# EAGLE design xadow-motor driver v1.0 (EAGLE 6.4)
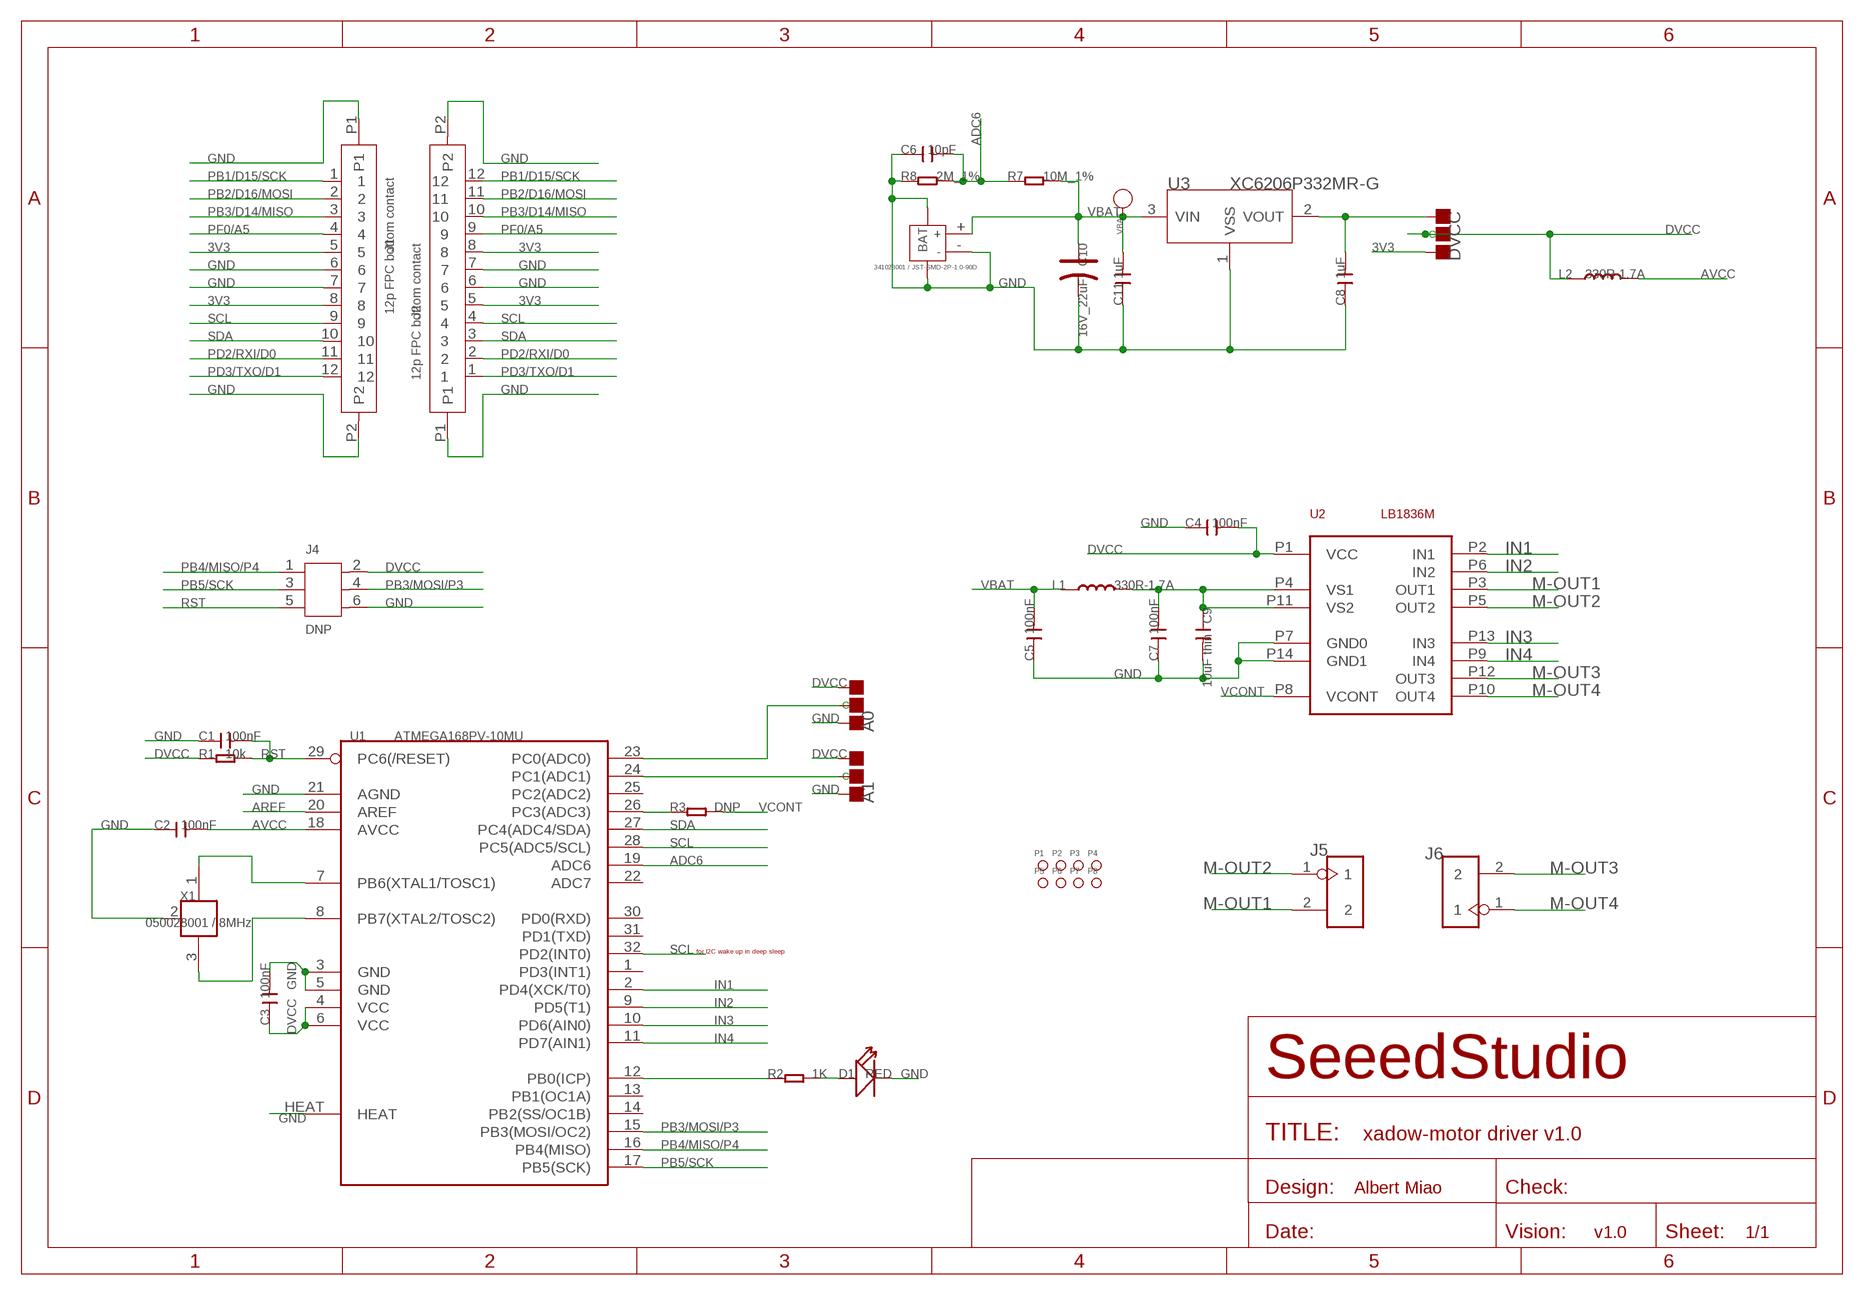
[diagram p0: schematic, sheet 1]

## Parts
A0  DNP  PAD-JUMPER-3P-40*40  [3P-SMD-4.1X1.5]
A1  DNP  PAD-JUMPER-3P-40*40  [3P-SMD-4.1X1.5]
BAT  341023001 / JST-SMD-2P-1.0-90D  JACK-JST-2P-SMD-PW'1.0'  [JST-SMD-2P-1.0-90D]
C1  100nF  C-0603  [C0603]
C2  100nF  C-0603  [C0603]
C3  100nF  C-0603  [C0603]
C4  100nF  C-0603  [C0603]
C5  100nF  C-0603  [C0603]
C6  10pF  C-0603  [C0603]
C7  100nF  C-0603  [C0603]
C8  1uF  C-0603  [C0603]
C9  10uF thin  C-0805  [C0805]
C10  16V_22uF  CAP-AVX-A  [AVX-A]
C11  1uF  C-0603  [C0603]
D1  RED  LED'0603'  [LED-0603]
DVCC  DNP  PAD-JUMPER-3P-40*40  [3P-SMD-4.1X1.5]
J1  12p FPC bottom contact  FPC052002-12LT  [12P-0.5]
J2  12p FPC bottom contact  FPC052002-12LT  [12P-0.5]
J4  DNP  HEADER-2X3P-1.27  [2X3P-1.27]
J5  HEADER-2P-2.0  [2P-2.0]
J6  HEADER-2P-2.0  [2P-2.0]
L1  330R-1.7A  L'0603'  [L0603]
L2  330R-1.7A  L'0603'  [L0603]
P1  PAD-MARK  [ROUND-MARK-1.0]
P2  PAD-MARK  [ROUND-MARK-1.0]
P3  PAD-MARK  [ROUND-MARK-1.0]
P4  PAD-MARK  [ROUND-MARK-1.0]
P5  PAD-MARK  [ROUND-MARK-1.0]
P6  PAD-MARK  [ROUND-MARK-1.0]
P7  PAD-MARK  [ROUND-MARK-1.0]
P8  PAD-MARK  [ROUND-MARK-1.0]
R1  10k  R-0603  [R0603]
R2  1K  R-0603  [R0603]
R3  DNP  R-0603  [R0603]
R7  10M_1%  R-0603  [R0603]
R8  2M_1%  R-0603  [R0603]
U1  ATMEGA168PV-10MU  MEGA8  [MLF32X]
U2  LB1836M  [MFP14S]
U3  XC6206P332MR-G  XC6206MR  [SOT23]
VBAT  PAD-TEST-POINT'4545'  [TP_4545]
X1  050028001 / 8MHz  XTAL_NCVER  [XTAL_3X2]

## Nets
3V3: DVCC.11(R) J1.5 J1.8 J2.5 J2.8
ADC6: C6.2 R7.1 R8.2 U1.19(ADC6)
AREF: U1.20(AREF)
AVCC: C2.2 L2.2 U1.18(AVCC)
DVCC [vcc]: A0.00(L) A1.00(L) C3.1 C4.2 DVCC.MM(C) J4.2 L2.1 R1.1 U1.4(VCC) U1.6(VCC) U2.P1(VCC)
GND: A0.11(R) A1.11(R) BAT.3 BAT.4 BAT.- C1.1 C2.1 C3.2 C4.1 C5.1 C6.1 C7.1 C8.1 C9.2 C10.- C11.1 D1.- J1.6 J1.7 J1.P1 J1.P2 J2.6 J2.7 J2.P1 J2.P2 J4.6 R8.1 U1.3(GND) U1.5(GND) U1.21(AGND) U1.HEAT U2.P7(GND0) U2.P14(GND1) U3.1(VSS) X1.2(GND)
IN1: U1.2(PD4(XCK/T0)) U2.P2(IN1)
IN2: U1.9(PD5(T1)) U2.P6(IN2)
IN3: U1.10(PD6(AIN0)) U2.P13(IN3)
IN4: U1.11(PD7(AIN1)) U2.P9(IN4)
M-OUT1 [HighCur]: J5.2 U2.P3(OUT1)
M-OUT2 [HighCur]: J5.1 U2.P5(OUT2)
M-OUT3 [HighCur]: J6.2 U2.P12(OUT3)
M-OUT4 [HighCur]: J6.1 U2.P10(OUT4)
N$2 [vcc]: C7.2 C9.1 L1.2 U2.P4(VS1) U2.P11(VS2)
N$3: R2.1 U1.12(PB0(ICP))
N$4: R3.1 U1.26(PC3(ADC3))
N$6: C8.2 DVCC.00(L) U3.2(VOUT)
N$7: A0.MM(C) U1.23(PC0(ADC0))
N$8: A1.MM(C) U1.24(PC1(ADC1))
N$9: D1.+ R2.2
N$22: U1.7(PB6(XTAL1/TOSC1)) X1.1
N$26: U1.8(PB7(XTAL2/TOSC2)) X1.3
PB1/D15/SCK: J1.1 J2.12
PB2/D16/MOSI: J1.2 J2.11
PB3/D14/MISO: J1.3 J2.10
PB3/MOSI/P3: J4.4 U1.15(PB3(MOSI/OC2))
PB4/MISO/P4: J4.1 U1.16(PB4(MISO))
PB5/SCK: J4.3 U1.17(PB5(SCK))
PD2/RXI/D0: J1.11 J2.2
PD3/TXO/D1: J1.12 J2.1
PF0/A5: J1.4 J2.9
RST: C1.2 J4.5 R1.2 U1.29(PC6(/RESET))
SCL: J1.9 J2.4 U1.28(PC5(ADC5/SCL)) U1.32(PD2(INT0))
SDA: J1.10 J2.3 U1.27(PC4(ADC4/SDA))
VBAT [vcc]: BAT.+ C5.2 C10.+ C11.2 L1.1 R7.2 U3.3(VIN) VBAT.T
VCONT: R3.2 U2.P8(VCONT)
Unconnected: U1.1(PD3(INT1)) U1.13(PB1(OC1A)) U1.14(PB2(SS/OC1B)) U1.22(ADC7) U1.25(PC2(ADC2)) U1.30(PD0(RXD)) U1.31(PD1(TXD))

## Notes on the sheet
- for I2C wake up in deep sleep
- Albert Miao
- v1.0

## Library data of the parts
A0 A1 DVCC = Discrete:PAD-JUMPER-3P; PARTNO: DNP
BAT = Connector :JACK-JST-2P-SMD-PW
C1-C9 C11 = Discrete:C*: Ceramic Capacitors
C10 = Discrete:CAP*: Electrolytic Capacitors,Tantalum Capacitors and Super Capacitors
D1 = Discrete:LED*
J1 J2 = template:FPC052002-12LT
J4 = template:HEADER-2X3P-1.27
J5 J6 = Connector:HEADER-2P
L1 L2 = Discrete:L*
P1-P8 = Discrete:PAD-MARK; PARTNO: DNP
R1-R3 R7 R8 = Discrete:R*
U1 = ICs_v54:MEGA8
U2 = LeoBuild:LB1836M
U3 = IC:XC6206: LOW ESR Cap.Compatible Positive Voltage Regulators
VBAT = Discrete:PAD-TEST-POINT; PARTNO: DNP
X1 = CPT_SMD:XTAL_NC

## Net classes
0 default: width 0.152 mm, drill 0.305 mm, clearance 0.152 mm
1 vcc: width 0.203 mm
2 HighCur: width 0.203 mm

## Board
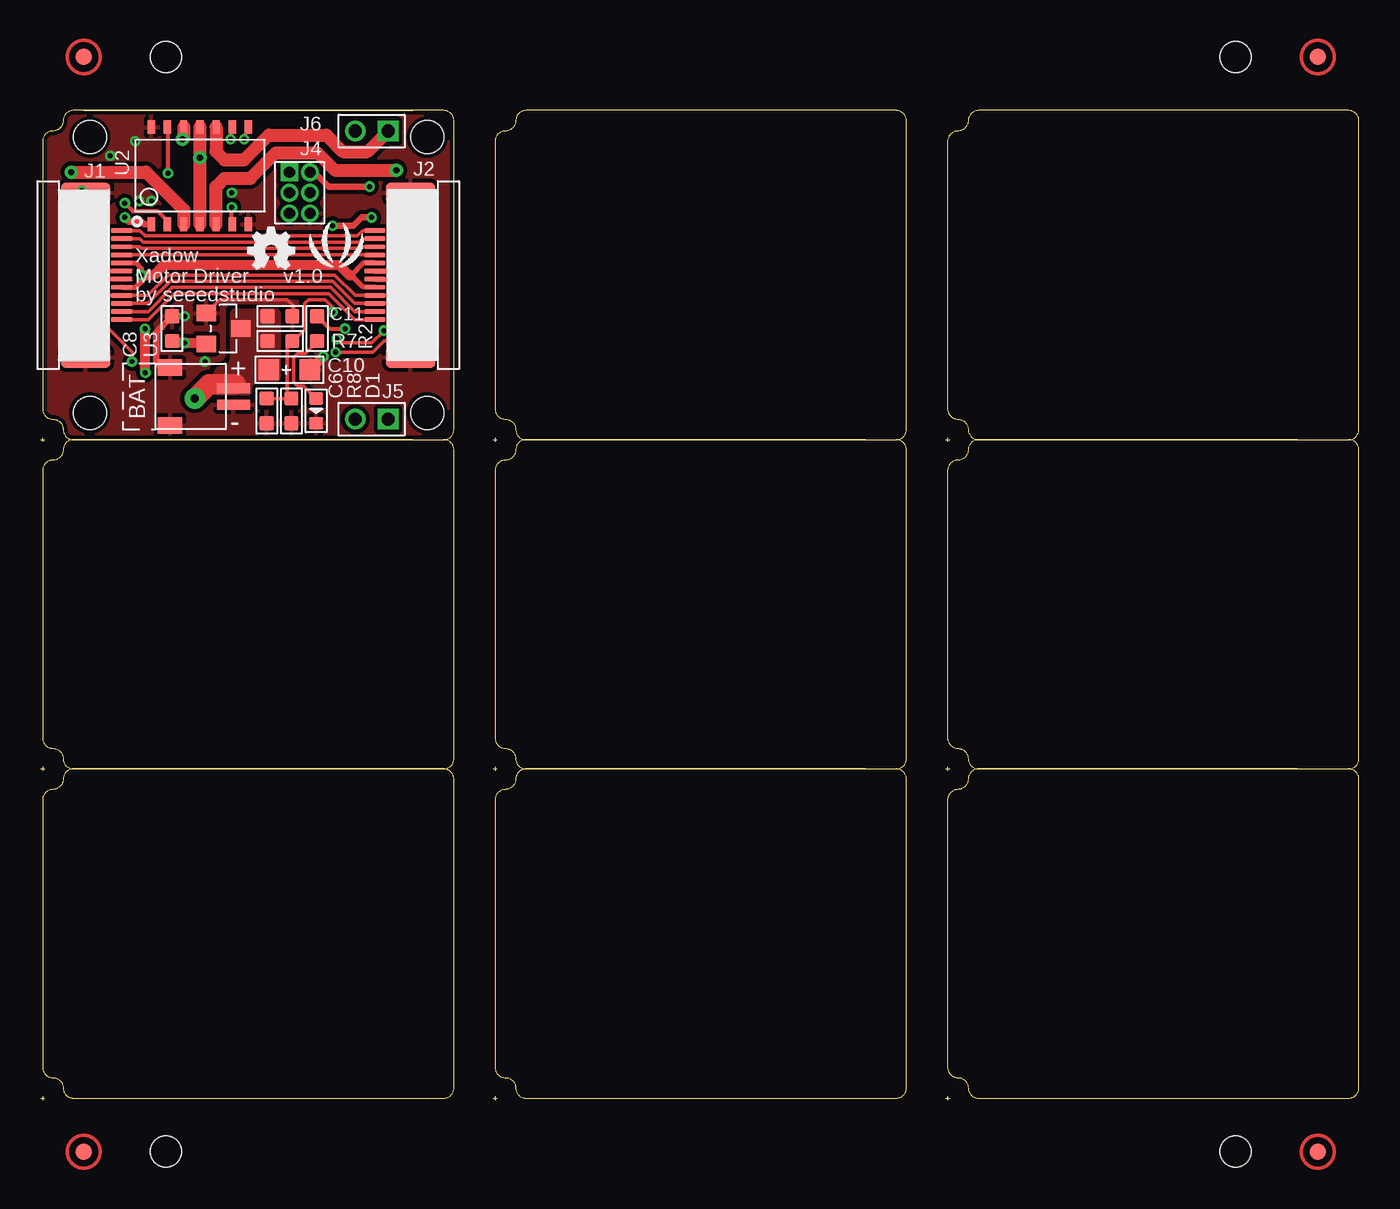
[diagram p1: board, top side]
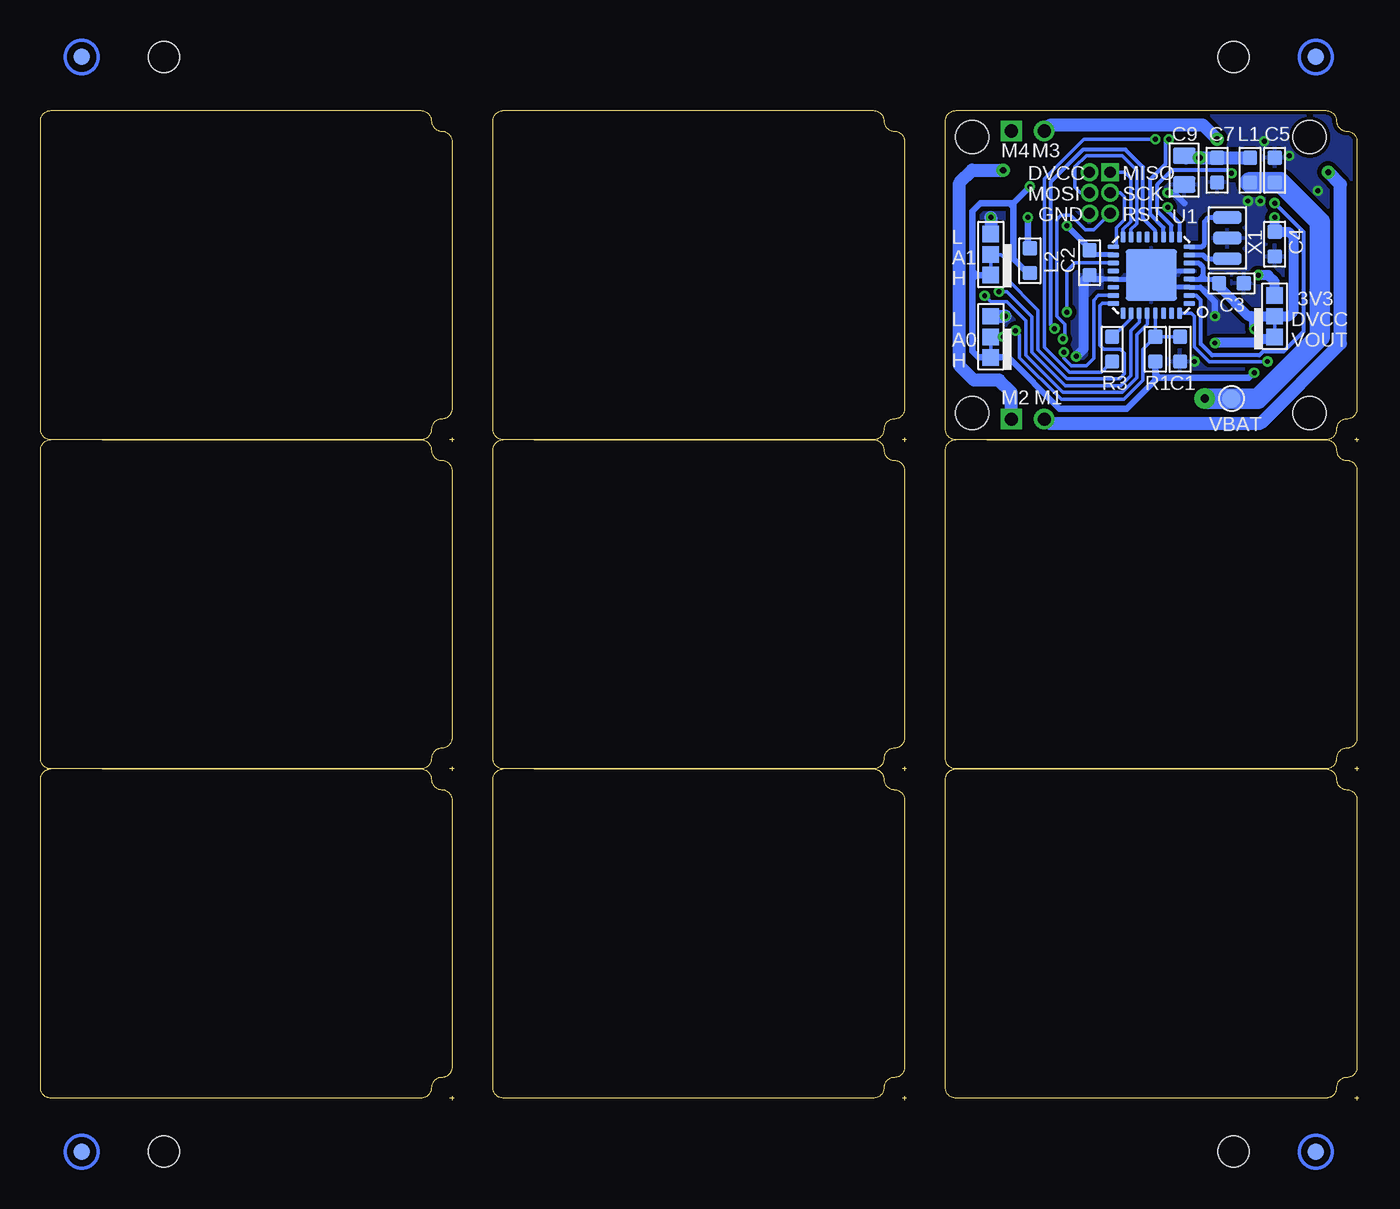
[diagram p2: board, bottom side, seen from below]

Size 81.41 x 61.09 mm. Coordinates in mm from the lower left corner, seen from the top.
Outline: 161 segments
Copper layers (1*16): Top 0.035mm / dielectric 1.5mm / Bottom 0.035mm
Design rules "SeeedStudio_rule_no_angle_090911 *": minimum track width 6mil, minimum drill 12mil, track to track 6mil, track to pad 6mil, pad to pad 6mil, via to via 6mil, smd to smd 0mil, copper to edge 10mil, drill to drill 10mil, minimum pad ring 6mil, minimum via ring 6mil, stop-mask expansion 2mil, vias tented up to drill 25mil, thermal gap 10mil
Holes 2.03 mm at 3.05,42.42 3.05,59.44 23.88,59.44 23.88,42.42
Holes 1.91 mm at 73.79,64.39 7.75,64.39 7.75,-3.17 73.79,-3.17
tRestrict: area 20,50.9 to 21.3,51; area 4.4,50.9 to 5.7,51; 12 lines
bRestrict: 12 lines

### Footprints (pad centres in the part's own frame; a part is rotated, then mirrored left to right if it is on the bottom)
3P-SMD-4.1X1.5 = smd 1.016 x 1.016: 00 -1.27,0; 11 1.27,0; MM 0,0
JST-SMD-2P-1.0-90D = smd 1.524 x 1.016: 3 -3.429,1.778; 4 -3.429,-1.778 | smd 2.032 x 0.635: + 0.508,0.508; - 0.508,-0.508
C0603 = smd 0.889 x 0.889: 1 -0.762,0; 2 0.762,0
C0805 = smd 1.016 x 1.397: 1 -0.889,0; 2 0.889,0
AVX-A = smd 1.27 x 1.27: + -1.27,0; - 1.27,0
LED-0603 = smd 0.762 x 0.889: + -0.762,0; - 0.762,0
12P-0.5 = smd 0.3 x 1.3: 1 -2.75,2.35; 2 -2.25,2.35; 3 -1.75,2.35; 4 -1.25,2.35; 5 -0.75,2.35; 6 -0.25,2.35; 7 0.25,2.35; 8 0.75,2.35; 9 1.25,2.35; 10 1.75,2.35; 11 2.25,2.35; 12 2.75,2.35 | smd 1.27 x 3.048: P1 -5.08,0.127; P2 5.08,0.127
2X3P-1.27 = drill 0.686 pad 1.092 square: 1 -0.635,1.27 | drill 0.686 pad 1.092: 2 0.635,1.27; 3 -0.635,0; 4 0.635,0; 5 -0.635,-1.27; 6 0.635,-1.27
2P-2.0 = drill 0.813 pad 1.27 square: 1 -1.016,0 | drill 0.813 pad 1.27: 2 1.016,0
L0603 = smd 0.889 x 0.889: 1 -0.762,0; 2 0.762,0
ROUND-MARK-1.0 = smd 1.016 x 1.016: P$1 0,0
R0603 = smd 0.889 x 0.889: 1 -0.762,0; 2 0.762,0
MLF32X = smd 0.7 x 0.3: 1 -2.35,1.75; 2 -2.35,1.25; 3 -2.35,0.75; 4 -2.35,0.25; 5 -2.35,-0.25; 6 -2.35,-0.75; 7 -2.35,-1.25; 8 -2.35,-1.75; 17 2.35,-1.75; 18 2.35,-1.25; 19 2.35,-0.75; 20 2.35,-0.25; 21 2.35,0.25; 22 2.35,0.75; 23 2.35,1.25; 24 2.35,1.75 | smd 0.3 x 0.7: 9 -1.75,-2.35; 10 -1.25,-2.35; 11 -0.75,-2.35; 12 -0.25,-2.35; 13 0.25,-2.35; 14 0.75,-2.35; 15 1.25,-2.35; 16 1.75,-2.35; 25 1.75,2.35; 26 1.25,2.35; 27 0.75,2.35; 28 0.25,2.35; 29 -0.25,2.35; 30 -0.75,2.35; 31 -1.25,2.35; 32 -1.75,2.35 | smd 3.175 x 3.175: HEAT 0,0
MFP14S = smd 0.45 x 0.85: P1 1,-0.8; P2 2,-0.8; P3 3,-0.8; P4 4,-0.8; P5 5,-0.8; P6 6,-0.8; P7 7,-0.8; P8 7,5.2; P9 6,5.2; P10 5,5.2; P11 4,5.2; P12 3,5.2; P13 2,5.2; P14 1,5.2
SOT23 = smd 1.016 x 1.2: 1 -0.95,-1.06; 2 0.95,-1.06; 3 0,1.06
TP_4545 = smd 1.143 x 1.143: T 0,0
XTAL_3X2 = smd 0.762 x 1.778: 1 -1.27,0; 2 0,0; 3 1.27,0

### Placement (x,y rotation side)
A0  22.73,47.12 90 bottom
A1  22.73,52.2 90 bottom
BAT  11.43,43.43 0 top
C1  11.05,46.35 90 bottom
C2  16.64,51.69 90 bottom
C3  7.87,50.42 0 bottom
C4  5.21,52.83 90 bottom
C5  5.21,57.4 270 bottom
C6  13.97,42.55 90 top
C7  8.76,57.4 90 bottom
C8  8.13,47.62 270 top
C9  10.79,57.4 270 bottom
C10  15.37,45.09 0 top
C11  14.8,48.39 180 top
D1  17.02,42.55 270 top
DVCC  5.21,48.39 90 bottom
J1  2.67,50.93 270 top
J2  22.99,50.93 90 top
J4  16,56.01 0 top
J5  20.45,42.04 180 top
J6  20.45,59.82 180 top
L1  6.73,57.4 90 bottom
L2  20.32,51.82 90 bottom
P1  not placed on the board
P2  not placed on the board
P3  not placed on the board
P4  not placed on the board
P5  not placed on the board
P6  not placed on the board
P7  not placed on the board
P8  not placed on the board
R1  12.57,46.35 90 bottom
R2  17.08,47.62 270 top
R3  15.24,46.35 270 bottom
R7  14.8,46.86 180 top
R8  15.49,42.55 90 top
U1  12.83,50.93 180 bottom
U2  5.84,54.86 0 top
U3  11.3,47.62 270 top
U$2  [SMALL_SEEED_LOGO]  18.29,52.96 0 top
U$3  [OSHW_FILLX100_NOTEXT]  12.83,51.31 0 top
VBAT  7.87,43.31 0 bottom
X1  8.13,53.21 90 bottom

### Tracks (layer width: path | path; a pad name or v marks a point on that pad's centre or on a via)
3V3  (via drill 0.3 pad 0.64)
  Top 0.305: J1.8 5.87,50.18 6.22,50.53 v6.22,50.93 6.22,51.33 5.87,51.68 J1.5 | J2.8 19.93,51.68 19.18,50.93 19.93,50.18 J2.5
  Top 0.61: v6.22,50.93 6.99,50.93 7.62,51.56 18.41,51.56 19.05,50.93 19.18,50.93
  Bottom 0.61: DVCC.11 5.21,50.55 5.59,50.93 v6.22,50.93
ADC6  (via drill 0.3 pad 0.64)
  Top 0.203: C6.2 R8.2 15.49,43.43 15.24,43.69 15.24,46.55 R7.1 15.62,46.86 16.32,47.56 16.32,49.17 16.55,49.4 17.58,49.4 18.03,48.95 v18.03,48.64
  Bottom 0.203: U1.19 17.54,51.68 18.03,51.18 v18.03,48.64
AVCC  (via drill 0.3 pad 0.64)
  Top 0.406: v18.03,53.98 19.3,53.98 19.81,54.48 v20.45,54.48
  Bottom 0.305: U1.18 16.36,52.18 C2.2
  Bottom 0.406: C2.2 16.64,52.58 v18.03,53.98 | v20.45,54.48 20.45,52.7 L2.2
DVCC  (via drill 0.3 pad 0.64)
  Top 0.406: J4.2 16.89,57.28 17.78,56.39 v20.32,56.39 | U2.P1 6.39,54.06 6.22,54.23 5.46,54.23 v5.21,54.48
  Top 0.61: v6.45,47.6 6.44,47.59 6.44,44.93 v6.48,44.89
  Bottom 0.203: A0.00 22.73,47.12 | A1.00 22.73,52.2 | DVCC.MM 5.21,47.12
  Bottom 0.254: 9.4,50.67 9.65,50.93 9.91,50.67
  Bottom 0.305: 10.02,51.68 U1.6 9.89,51.68 9.65,51.44 9.65,50.93 9.65,50.68 | U1.4 9.65,50.68 | 9.65,50.68 8.89,50.68 C3.1
  Bottom 0.406: R1.1 12.57,44.83 | 12.57,44.83 12.57,44.58 | 12.57,44.58 12.57,44.45 14.34,42.69 18.49,42.69 21.65,45.85 A0.00 23.49,45.85 23.88,46.23 23.88,50.67 | 12.57,44.58 12.32,44.58 | L2.1 20.45,51.05 21.34,51.94 21.34,55.12 | 23.88,50.67 23.88,50.93 | 23.88,50.93 23.88,51.18 | 23.88,51.18 23.88,54.86 23.37,55.37 21.59,55.37 | 21.34,55.12 21.34,55.37 | 21.34,55.37 v20.32,56.39 | 21.59,55.37 21.34,55.37 | 21.59,55.37 21.34,55.12 | A1.00 23.62,50.93 | 23.62,50.93 23.88,50.93 | 12.32,44.58 12.57,44.83 | 12.32,44.58 6.79,44.58 v6.48,44.89 | 23.62,50.93 23.88,51.18 | 23.62,50.93 23.88,50.67
  Bottom 0.61: DVCC.MM 5.32,48.39 5.33,48.39 | v5.21,54.48 C4.2 4.35,53.59 4.06,53.31 4.06,48.64 4.32,48.39 DVCC.MM | C3.1 8.64,50.19 6.83,48.39 6.67,48.39 | 6.67,48.39 6.35,48.39 | 6.35,48.39 6.22,48.39 | 6.22,48.39 5.33,48.39 DVCC.MM | v6.45,47.6 6.45,48.16 | 6.45,48.17 6.45,48.28 6.35,48.39 | 6.45,48.16 6.22,48.39 | 6.45,48.16 6.45,48.17 | 6.45,48.17 6.67,48.39
GND  (via drill 0.3 pad 0.64)
  Top 0.203: U3.1 11.07,49.4 15.24,49.4 15.62,49.02 15.62,48.45 C11.1
  Top 0.305: J1.6 3.18,51.18 | J1.7 3.18,50.68 3.18,50.67 | J2.6 21.47,50.68 21.84,51.05 22.73,51.05 | J2.7 21.33,51.18 21.72,51.56 22.61,51.56
  Top 0.406: 7.62,45.09 7.15,45.56 7.15,47.41 C8.1
  Top 0.61: C10.- 16.76,45.09 16.76,45.21 17.4,45.85
  Bottom 0.305: 15.87,50.68 U1.21 12.95,50.68 12.83,50.8 | 12.83,50.8 12.83,50.55 12.46,50.18 U1.3 9.79,50.18 9.53,49.91 | 12.83,50.8 U1.HEAT 12.83,51.18 12.82,51.18 U1.5
  Bottom 0.406: 15.87,50.68 16.39,50.68 C2.1 | 9.53,49.91 8.89,49.28 v8.89,48.39 | v11.81,56.01 11.43,56.01 10.79,55.37
  Bottom 0.61: C2.1 17.02,50.55 17.02,46.35 v17.46,45.91
  Bottom 0.813: A0.11 v21.84,48.39 | v22.73,54.48 A1.11
  other vias: 10.16,45.59 5.84,59.18 4.32,58.29 6.1,55.5 6.86,55.5 2.54,56.13
  pour Top (isolate 0.254, rank 2): 0.13,61.09 25.53,61.09 25.53,40.77 0.13,40.77
  pour Bottom (isolate 0.254, rank 2): 0.13,61.09 25.53,61.09 25.53,40.77 0.13,40.77
IN1  (via drill 0.3 pad 0.64)
  Top 0.254: U2.P2 7.84,54.26 7.24,54.86 5.71,54.86 v5.21,55.37
  Bottom 0.254: U1.2 10.07,49.68 9.78,49.38 9.78,46.69 9.07,45.97 6.16,45.97 5.93,46.21 4.66,46.21 3.43,47.44 3.43,53.59 v5.21,55.37
IN2  (via drill 0.3 pad 0.64)
  Top 0.203: 11.81,54.09 U2.P6
  Top 0.254: 11.81,54.09 v11.81,55.12
  Bottom 0.254: U1.9 11.08,54.13 11.81,54.86 v11.81,55.12
IN3  (via drill 0.3 pad 0.64)
  Top 0.254: U2.P13 7.84,57.25 v7.87,57.21
  Bottom 0.254: U1.10 11.58,53.99 12.44,54.85 12.44,56.52 11.56,57.4 8.06,57.4 v7.87,57.21
IN4  (via drill 0.3 pad 0.64)
  Top 0.203: v11.75,59.31 11.75,59.97 U2.P9
  Bottom 0.254: U1.11 12.08,53.86 12.89,54.67 12.89,56.83 11.94,57.78 11.94,59.12 v11.75,59.31
M-OUT1  (via drill 0.38 pad 0.81)
  Top 0.813: v1.9,57.28 6.52,57.28 8.84,54.95 U2.P3
  Bottom 0.813: J5.2 19.18,41.78 6.07,41.78 1.14,46.71 1.14,56.52 v1.9,57.28
M-OUT2  (via drill 0.38 pad 0.81)
  Top 0.813: U2.P5 10.84,56.39 11.35,56.9 12.95,56.9 14.53,58.48 17.09,58.48 18.16,57.4 v21.97,57.4
  Bottom 0.813: v21.97,57.4 23.88,57.4 24.67,56.61 24.67,45.35 23.77,44.45 22.23,44.45 21.46,43.69 J5.1
M-OUT3  (via drill 0.38 pad 0.81)
  Top 0.813: U2.P12 8.84,59.39 v8.76,59.31
  Bottom 0.813: v8.76,59.31 9.65,60.2 19.05,60.2 J6.2
M-OUT4
  Top 0.813: U2.P10 10.84,58.55 11.35,58.04 12.57,58.04 14.1,59.56 17.65,59.56 18.67,58.55 20.19,58.55 J6.1
N$2  (via drill 0.38 pad 0.81)
  Top 0.813: U2.P11 v9.84,58.17 U2.P4
  Bottom 0.813: L1.2 C7.2 v9.84,58.17 10.67,58.17 C9.1
N$3  (via drill 0.3 pad 0.64)
  Top 0.203: R2.1 17.27,48.39
  Top 0.254: R2.1 17.84,47.62 v18.8,47.62
  Bottom 0.254: U1.12 12.58,53.66 13.34,54.42 13.34,57.6 14.41,58.67 17.04,58.67 19.05,56.66 19.05,47.88 v18.8,47.62
N$4
  Bottom 0.203: R3.1 15.19,47.12 14.08,48.23 U1.26
N$6  (via drill 0.3 pad 0.64)
  Top 0.61: 10.24,46.53 U3.2 10.18,46.74 v8.89,46.74 8.25,46.74 C8.2
  Bottom 0.61: v8.89,46.74 6.22,46.74 5.97,46.99 5.33,46.99 DVCC.00
N$7  (via drill 0.3 pad 0.64)
  Top 0.203: v21.97,47.12 21.72,46.86 21.21,46.86 20.51,46.16 v18.22,46.16
  Bottom 0.203: v21.97,47.12 A0.MM | U1.23 16.09,49.68 16.38,49.38 16.38,45.79 16.85,45.33 17.77,45.33 18.22,45.78 v18.22,46.16
N$8
  Bottom 0.203: A1.MM 22.1,52.2 21.84,51.94 21.84,50.8 19.81,48.77 19.81,46.32 18.03,44.53 14.78,44.53 14.48,44.83 14.48,46.1 14.73,46.35 15.75,46.35 16,46.61 16,49.02 15.85,49.18 U1.24
N$9
  Top 0.203: D1.+ 16.26,44.07 15.88,44.07 15.62,44.32 15.62,45.85 15.88,46.1 16.38,46.1 17.02,46.74 17.02,46.8 R2.2
N$22
  Bottom 0.305: U1.7 9.63,52.18 9.4,51.94 X1.1
N$26
  Bottom 0.305: U1.8 9.68,52.68 9.53,52.83 9.53,54.23 9.27,54.48 X1.3
PB1/D15/SCK
  Top 0.203: J1.1 6.14,53.68 6.48,53.34 19.56,53.34 19.89,53.68 J2.12
PB2/D16/MOSI
  Top 0.203: J1.2 6.13,53.18 6.35,52.96 19.68,52.96 19.9,53.18 J2.11
PB3/D14/MISO
  Top 0.203: J1.3 6.12,52.68 6.22,52.58 19.81,52.58 19.91,52.68 J2.10
PB3/MOSI/P3
  Bottom 0.203: U1.15 14.08,53.74 13.72,54.1 13.72,57.4 14.61,58.29 16.84,58.29 17.53,57.6 17.53,56.34 17.2,56.01 J4.4
PB4/MISO/P4
  Bottom 0.203: U1.16 14.58,53.75 14.1,54.23 14.1,56.9 14.48,57.28 J4.1
PB5/SCK
  Bottom 0.203: J4.3 14.73,56.01 14.48,55.75 14.48,54.36 14.99,53.85 14.99,52.87 U1.17
PD2/RXI/D0
  Top 0.203: J1.11 6.64,48.68 8.13,50.16 17.91,50.16 19.39,48.68 J2.2
PD3/TXO/D1
  Top 0.203: J1.12 6.65,48.18 8.25,49.78 17.78,49.78 19.39,48.18 J2.1
PF0/A5
  Top 0.203: J1.4 J2.9
RST  (via drill 0.3 pad 0.64)
  Top 0.203: v18.29,46.99 18.54,46.74 20.45,46.74 v21.21,47.5
  Bottom 0.203: C1.2 R1.2 | R1.2 13.34,46.35 13.34,44.45 14.53,43.26 18.38,43.26 20.95,45.83 20.95,47.24 v21.21,47.5 | U1.29 R1.2 | J4.5 16.38,53.72 16.89,53.72 17.78,54.61 18.41,54.61 18.67,54.36 18.67,48.39 18.16,47.88 18.16,47.12 v18.29,46.99
SCL  (via drill 0.3 pad 0.64)
  Top 0.203: v23.11,49.66 23.11,50.19 22.76,50.55 21.95,50.55 21.59,50.19 21.59,49.84 21.42,49.68 J2.4 19.41,49.68 18.16,50.93 7.87,50.93 6.62,49.68 J1.9 4.21,49.68 3.99,49.45 3.99,47.83 5.65,46.16 v5.65,45.59
  Bottom 0.203: U1.32 10.35,48.58 10.16,48.39 10.16,46.51 9.24,45.59 v5.65,45.59 | U1.28 13.08,47.88 13.72,47.24 13.72,44.58 14.6,43.69 18.29,43.69 20.57,45.98 20.57,48.09 21.76,49.28 22.73,49.28 v23.11,49.66
SDA  (via drill 0.3 pad 0.64)
  Top 0.203: v22.23,49.91 21.49,49.18 J2.3 19.4,49.18 18.03,50.55 8,50.55 6.63,49.18 J1.10
  Bottom 0.203: U1.27 13.58,48.02 14.1,47.5 14.1,44.7 14.71,44.09 18.13,44.09 20.19,46.16 20.19,48.36 21.74,49.91 v22.23,49.91
VBAT  (via drill 0.51 pad 1.27)
  Top 0.406: 12.06,44.2 12.06,44.07 BAT.+
  Top 1.27: 12.06,44.2 10.41,44.2 v9.53,43.31
  Bottom 1.27: v9.53,43.31 VBAT.T 6.25,43.31 2.42,47.14 2.42,54.21 4.85,56.64 C5.2 L1.1
  pour Top (isolate 0.254, no thermals): 10.79,44.83 10.79,43.81 arc90 11.05,43.56 12.7,43.56 arc90 12.95,43.81 arc-90 13.59,44.45 14.48,44.45 arc90 14.73,44.7 14.73,48.51 arc90 14.48,48.77 12.06,48.77 arc90 11.81,48.51 11.81,45.85 arc-90 11.18,45.21 arc90
VCONT  (via drill 0.3 pad 0.64)
  Top 0.203: v12.57,59.31 12.57,59.56 12.83,59.82 12.83,60.05 U2.P8
  Bottom 0.203: v12.57,59.31 16.99,59.31 19.43,56.87 19.43,46.48 17.87,44.92 15.91,44.92 R3.2

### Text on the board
tPlace: Xadow | Motor Driver | v1.0 | by seeedstudio | + | -
bPlace: M3 | M4 | MISO | DVCC | SCK | MOSI | RST | GND | L | H | 3V3 | L | VOUT | H | M1 | M2
tEnhance: Top Enhance 0.25~0.28mm
bEnhance: Bottom Enhance
bEnHoles: Holes on Bottom Enhance | All Holes are 70mil diameter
